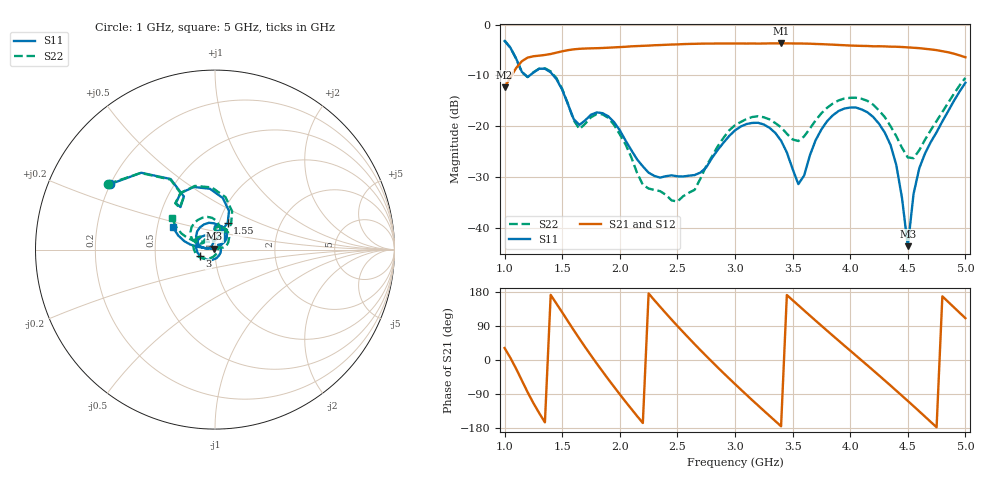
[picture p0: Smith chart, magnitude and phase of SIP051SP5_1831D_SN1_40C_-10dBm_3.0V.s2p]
# GHz  S  dB  R  50
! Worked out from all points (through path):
!   81 points, 1 GHz to 5 GHz, reference 50 ohm
!   highest |S21| = -3.68 dB at 3.4 GHz (marker M1); lowest = -12.3 dB at 1 GHz (marker M2)
!   lowest |S11| = -43.6 dB at 4.5 GHz (marker M3), VSWR 1.01, Z = 49.7 + j0.582 ohm
!   |S11| at or under -10 dB: 1.185 GHz to 1.217 GHz (32.19 MHz wide, 2.68 % of centre); 1.423 GHz to end of sweep
!   |S22| runs from -34.8 to -3.1 dB; largest |S21 - S12| = 0.0037
!   S11 on the Smith chart (normalised r, x): 1 GHz: 0.20, +0.27; 1.55 GHz: 1.10, +0.34; 3 GHz: 0.84, -0.06; 5 GHz: 0.60, +0.16
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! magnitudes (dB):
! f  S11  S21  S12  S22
! 1 GHz  -3.2  -12.3  -12.3  -3.1
! 1.2 GHz  -10.3  -6.5  -6.5  -10.3
! 1.4 GHz  -9.4  -5.8  -5.8  -9.2
! 1.55 GHz  -15.7  -5.0  -5.0  -15.6
! 1.65 GHz  -19.7  -4.8  -4.8  -20.5
! 1.7 GHz  -18.8  -4.7  -4.7  -19.5
! 1.9 GHz  -18.0  -4.5  -4.5  -18.3
! 2.2 GHz  -27.9  -4.2  -4.2  -31.5
! 2.35 GHz  -30.1  -4.0  -4.0  -32.7
! 2.65 GHz  -29.6  -3.8  -3.8  -32.5
! 3 GHz  -20.8  -3.7  -3.7  -19.8
! 3.2 GHz  -19.3  -3.7  -3.7  -18.0
! 3.4 GHz  -22.8  -3.7  -3.7  -20.2
! 3.55 GHz  -31.4  -3.7  -3.7  -22.9
! 3.7 GHz  -22.7  -3.8  -3.8  -18.8
! 4.05 GHz  -16.3  -4.1  -4.2  -14.4
! 4.35 GHz  -23.6  -4.3  -4.3  -20.0
! 4.45 GHz  -34.1  -4.4  -4.4  -24.2
! 4.5 GHz  -43.6  -4.5  -4.5  -26.1
! 4.55 GHz  -33.3  -4.5  -4.5  -26.3
! 4.6 GHz  -28.2  -4.6  -4.6  -24.7
! 5 GHz  -11.4  -6.4  -6.4  -10.5
